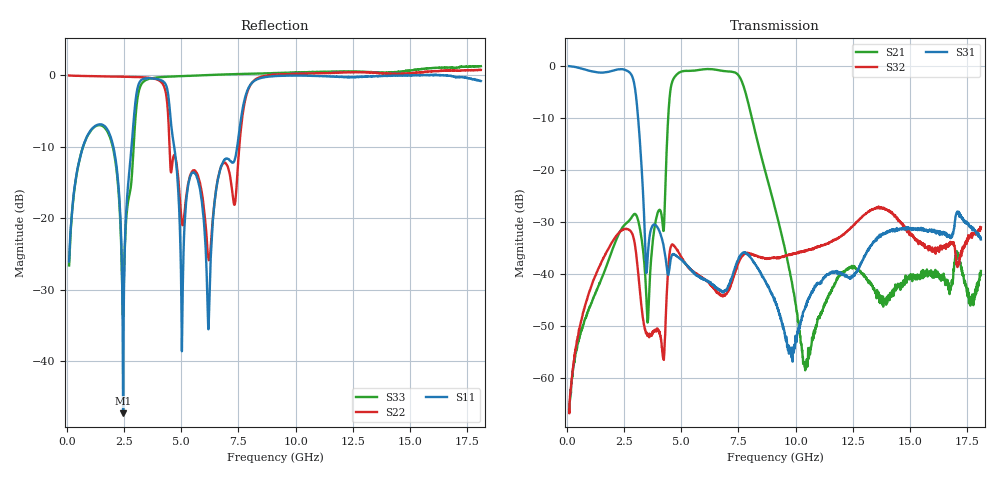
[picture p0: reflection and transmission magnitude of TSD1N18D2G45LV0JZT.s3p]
# MHZ S RI R 50
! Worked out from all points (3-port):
!   1801 points, 100 MHz to 18.1 GHz, reference 50 ohm
!   strongest paths, dB at 100 MHz, 4.6 GHz, 9.1 GHz, 13.6 GHz, 18.1 GHz:
!     S31: 0.0, -36.4, -45.3, -32.9, -33.3
!     S32: -66.1, -34.3, -36.9, -27.2, -31.1
!     S21: -66.4, -3.1, -27.3, -44.2, -39.4
!   lowest |S11| = -47.3 dB at 2.46 GHz (marker M1), VSWR 1.01, Z = 49.7 - j0.26 ohm
!   |S11| at or under -10 dB: start of sweep to 708.2 MHz; 2.031 GHz to 2.828 GHz (796.8 MHz wide, 32.8 % of centre); 4.692 GHz to 7.448 GHz (2.756 GHz wide, 45.4 % of centre)
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100  -0.00142 -0.0499  -7.45e-05 -0.00044  0.9908 -0.1046
     -4.61e-05 -0.000475  -0.9936 0.0206  2.18e-05 0.000446
     0.9904 -0.1033  3.26e-06 0.000496  -0.00232 -0.0466
1620  -0.444 -0.000578  -0.00959 -0.00364  0.00399 -0.8645
      -0.00956 -0.00376  -0.9457 0.2541  0.00507 0.0136
      0.004 -0.8652  0.0052 0.0136  -0.4326 -0.026
2460  -0.00343 -0.00262  -0.0281 0.00498  -0.8967 -0.2417
      -0.0282 0.00483  -0.8885 0.4001  0.0269 0.000277
      -0.8964 -0.2409  0.0267 0.000253  -0.0205 -0.00761
3500  -0.7933 -0.5236  -0.00289 0.0035  -0.00317 0.0105
      -0.00286 0.00355  -0.6156 0.7372  -0.00129 0.00228
      -0.00322 0.0105  -0.0012 0.00238  0.2692 -0.8903
4880  -0.00378 0.1453  -0.8285 0.203  -0.0111 0.00934
      -0.8303 0.2063  -0.03 0.1806  0.00268 0.0161
      -0.0111 0.00938  0.00261 0.0161  -0.5758 -0.7944
6430  0.0748 -0.089  0.9092 0.1718  0.00637 0.00443
      0.9118 0.1688  -0.0681 -0.0982  0.00716 0.0013
      0.00632 0.00444  0.00715 0.00122  -0.7996 -0.6073
7400  0.1033 -0.2624  0.1577 -0.8348  0.00889 0.00844
      0.1563 -0.84  0.0693 0.1336  -0.00242 -0.0108
      0.00911 0.00851  -0.00258 -0.0109  -0.8266 -0.5914
9100  -0.6133 -0.77  -0.0399 0.0143  0.00493 -0.00214
      -0.0408 0.0145  -0.2359 -0.9798  -0.0126 0.00721
      0.00497 -0.00213  -0.0125 0.00704  -0.8335 -0.6128
10430  -0.887 -0.4431  0.000305 0.00125  -0.000515 0.0049
       0.000232 0.00123  -0.4145 -0.9366  -0.0141 0.00932
       -0.000591 0.00488  -0.0138 0.00948  -0.8073 -0.6641
18100  -0.8744 0.2537  -0.00582 -0.00948  -0.00379 0.0217
       -0.00499 -0.00947  -0.7744 -0.7646  -0.026 0.00921
       -0.00406 0.0211  -0.0266 0.00873  -0.9204 -0.6961
